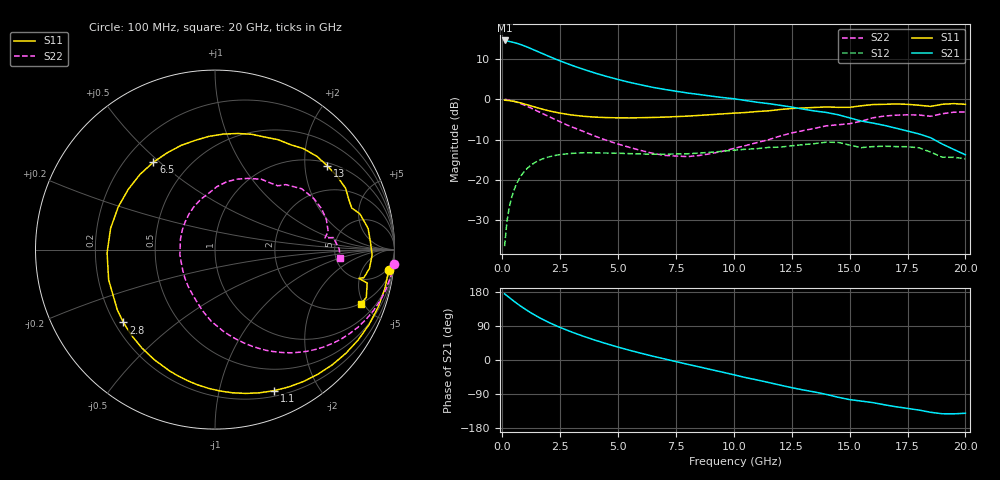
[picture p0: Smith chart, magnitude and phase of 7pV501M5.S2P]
! Infineon Technologies  Discrete & RF Semiconductors
! bfp620
! VCE = 0.50 V,  IC =  1.5 mA
! Common Emitter S-Parameters:  Sep 2002
# GHz  S  MA  R  50
!  f  S11  S21  S12  S22
! GHz  MAG  ANG  MAG  ANG  MAG  ANG  MAG  ANG
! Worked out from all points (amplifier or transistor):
!   59 points, 100 MHz to 20 GHz, reference 50 ohm
!   highest |S21| = 14.6 dB at 100 MHz (marker M1)
!   |S21| within 3 dB of that: start of sweep to 1.632 GHz
!   unconditionally stable (mu >= 1): 6.058 GHz to 13.51 GHz; 14.44 GHz to 15.75 GHz; 17.18 GHz to end of sweep
!   at 1 GHz: K = 0.16, MSG = 15.4 dB, |S12| = -17.6 dB
!   at 5.5 GHz: K = 0.91, MSG = 8.8 dB, |S12| = -13.5 dB
!   at 20 GHz: K = 2.08, MAG = -5.4 dB, |S12| = -14.7 dB
!   S11 on the Smith chart (normalised r, x): 100 MHz: 4, -16; 1.1 GHz: 0.26, -1.47; 2.8 GHz: 0.24, -0.33; 6.5 GHz: 0.32, +0.48; 13 GHz: 1.09, +2.61; 20 GHz: 1.99, -4.79
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0.1  0.9752 -6.7  5.37 174.4  0.0151 85.1  0.9987 -4.5
0.2  0.9707 -13.2  5.294 169.7  0.0304 81.7  0.9904 -8.8
0.3  0.9637 -19.6  5.22 164.9  0.0455 77.8  0.9785 -13.0
0.6  0.9303 -38.4  4.974 150.7  0.0874 66.1  0.9271 -24.8
0.8  0.9007 -50.4  4.769 141.9  0.1114 58.7  0.8839 -32.0
1.1  0.8519 -67.3  4.418 129.8  0.1412 48.6  0.8128 -41.9
1.5  0.7885 -87.9  3.947 115.2  0.1701 37.2  0.7177 -53.2
1.9  0.7336 -106.2  3.525 102.5  0.1892 27.8  0.6328 -62.7
2.4  0.6827 -126.7  3.071 88.5  0.2043 18.1  0.5427 -73.0
2.8  0.652 -141.5  2.778 78.6  0.2108 11.4  0.4803 -80.9
3.5  0.6161 -164.1  2.36 62.7  0.2175 1.5  0.3999 -93.0
4  0.6015 -178.3  2.119 52.4  0.2172 -4.4  0.3497 -101.1
5  0.5893 156.3  1.762 34.0  0.2142 -12.9  0.2788 -116.9
6.5  0.596 125.2  1.408 10.1  0.2085 -22.0  0.214 -146.9
7  0.6015 116.2  1.328 3.0  0.2085 -23.9  0.2018 -158.2
8.5  0.632 93.0  1.148 -18.1  0.2156 -29.6  0.2011 163.1
10.5  0.6858 66.1  0.968 -46.3  0.2402 -40.4  0.2664 116.0
13  0.7806 36.7  0.755 -79.1  0.2742 -57.5  0.4101 73.0
13.5  0.7936 31.0  0.716 -84.5  0.2827 -62.0  0.4375 65.1
15  0.7964 16.9  0.589 -104.5  0.2712 -82.7  0.4985 45.5
17  0.8759 -2.0  0.439 -123.3  0.2594 -94.7  0.6358 20.9
20  0.8665 -20.3  0.205 -140.5  0.1834 -117.0  0.6983 -3.9
